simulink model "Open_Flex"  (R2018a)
settings: Solver=VariableStepAuto  StartTime=0.0  StopTime=25  FixedStep=0.0001  RelTol=1e-5  EnableMultiTasking=on
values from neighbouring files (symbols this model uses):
  d2r = pi/180    (= 0.0174532925199)    [init.m]    (also in LQR_Design.m)
  Kr = Kq; Kr(3:4)=-Kq(3:4)    [init.m]
  Wf = 24    [init.m]
undefined symbols (not defined in the file or in its folder): Aa, Av, Ba, Bv, Ca, Cv, Da, Dv, Kq, TVC

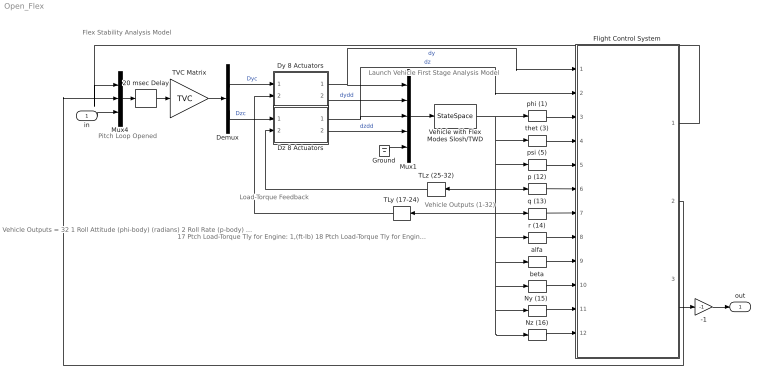
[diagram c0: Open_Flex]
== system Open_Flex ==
  note: Load-Torque Feedback
  note: 17 Ptch Load-Torque Tly for Engine: 1,(ft-lb) 18 Ptch Load-Torque Tly for Engine: 2,(ft-lb) 19 Ptch Load-Torque Tly for Engine: 3,(ft-lb) 20 Ptch Load-Torque Tly for Engine: 4,(ft-lb) 21 Ptch Load-Torque Tly for Engine: 5,(ft-lb) 22 Ptch Load-Torque Tly for Engine: 6,(ft-lb) 23 Ptch Load-Torque Tly for Engine: 7,(ft-lb) 24 Ptch Load-Torque Tly for Engine: 8,(ft-lb) 25 Yaw Load-Torque Tlz for Engine: 1,(ft-lb) 26 Yaw Load-Torque Tlz for Engine: 2,(ft-lb) 27 Yaw Load-Torque Tlz for Engine: 3,(ft-lb) 28 Yaw Load-Torque Tlz for Engine: 4,(ft-lb) 29 Yaw Load-Torque Tlz for Engine: 5,(ft-lb) 30 Yaw Load-Torque Tlz for Engine: 6,(ft-lb) 31 Yaw Load-Torque Tlz for Engine: 7,(ft-lb) 32 Yaw Load-Torque Tlz for Engine: 8,(ft-lb)
  note: Vehicle Outputs = 32 1 Roll Attitude (phi-body) (radians) 2 Roll Rate (p-body) (rad/sec) 3 Pitch Attitude (thet-bdy) (radians) 4 Pitch Rate (q-body) (rad/sec) 5 Yaw Attitude (psi-body) (radians) 6 Yaw Rate (r-body) (rad/sec) 7 Angle of attack, alfa, (radians) 8 Angle of sideslip, beta, (radian) 9 Change in Altitude, delta-h, (feet) 10 Forward Acceleration (V-dot) (ft/sec) 11 Cross Range Velocity (Vcr) (ft/sec) 12 Rate-Gyro # 1, Roll Rate (Body) (rad/sec) 13 Rate-Gyro # 2, Pitch Rate (Body) (rad/sec) 14 Rate-Gyro # 3, Yaw Rate (Body) (rad/sec) 15 Accelerom # 1, (along Y), (ft/sec^2) Translat. Accelerat. 16 Accelerom # 2, (along Z), (ft/sec^2) Translat. Accelerat.
  note: Vehicle Outputs (1-32)
  note: Flex Stability Analysis Model
  note: Pitch Loop Opened
  note: Launch Vehicle First Stage Analysis Model
  in : Inport
  -1 : Gain  Gain=-1
  20 msec Delay : TransportDelay  DelayTime="[1  1  1]*0.02"  InitialOutput="[0  0  0]"  PadeOrder=2
  Demux : Demux  Outputs=[8, 8]
  Dy 8 Actuators : Subsystem
  Dz 8 Actuators : Subsystem
  Flight Control System : Subsystem
  Ground : Ground
  Mux1 : Mux  Inputs=[8, 8, 8, 8, 1]
  Mux4 : Mux  Inputs=3
  "Ny (15) " : Selector  InputPortWidth=32  IndexOptions=Index vector (dialog)  Indices=[15]  OutputSizes=1
  Nz (16) : Selector  InputPortWidth=32  IndexOptions=Index vector (dialog)  Indices=[16]  OutputSizes=1
  TLy (17-24) : Selector  InputPortWidth=32  IndexOptions=Index vector (dialog)  Indices=[17:24]  OutputSizes=1
  TLz (25-32) : Selector  InputPortWidth=32  IndexOptions=Index vector (dialog)  Indices=[25:32]  OutputSizes=1
  TVC Matrix : Gain  Gain=TVC  Multiplication=Matrix(K*u)
  Vehicle with Flex Modes Slosh/TWD : StateSpace  A=Av  B=Bv  C=Cv  D=Dv  InitialCondition=0
  alfa : Selector  InputPortWidth=32  IndexOptions=Index vector (dialog)  Indices=[7]  OutputSizes=1
  beta : Selector  InputPortWidth=32  IndexOptions=Index vector (dialog)  Indices=[8]  OutputSizes=1
  p (12) : Selector  InputPortWidth=32  IndexOptions=Index vector (dialog)  Indices=[12]  OutputSizes=1
  phi (1) : Selector  InputPortWidth=32  IndexOptions=Index vector (dialog)  Indices=[1]  OutputSizes=1
  psi (5) : Selector  InputPortWidth=32  IndexOptions=Index vector (dialog)  Indices=[5]  OutputSizes=1
  q (13) : Selector  InputPortWidth=32  IndexOptions=Index vector (dialog)  Indices=[13]  OutputSizes=1
  r (14) : Selector  InputPortWidth=32  IndexOptions=Index vector (dialog)  Indices=[14]  OutputSizes=1
  thet (3) : Selector  InputPortWidth=32  IndexOptions=Index vector (dialog)  Indices=[3]  OutputSizes=1
  out : Outport
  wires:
  Mux1/1 -> Vehicle with Flex Modes Slosh/TWD/1
  Dy 8 Actuators/2(dydd) -> Mux1/2  "dydd"
  Dz 8 Actuators/2(dzdd) -> Mux1/4  "dzdd"
  Demux/1 -> Dy 8 Actuators/1(dyc)  "Dyc"
  Dy 8 Actuators/1(dy) -> Flight Control System/1(dy), Mux1/1  "dy"
  Dz 8 Actuators/1(dz) -> Flight Control System/2(dz), Mux1/3  "dz"
  Demux/2 -> Dz 8 Actuators/1(dzc)  "Dzc"
  TLy (17-24)/1 -> Dy 8 Actuators/2(TLy)
  TLz (25-32)/1 -> Dz 8 Actuators/2(TLz)
  Vehicle with Flex Modes Slosh/TWD/1 -> "Ny (15) "/1, Nz (16)/1, beta/1, alfa/1, r (14)/1, TLy (17-24)/1, q (13)/1, TLz (25-32)/1, p (12)/1, psi (5)/1, thet (3)/1, phi (1)/1
  r (14)/1 -> Flight Control System/8(r)
  q (13)/1 -> Flight Control System/7(q)
  p (12)/1 -> Flight Control System/6(p)
  alfa/1 -> Flight Control System/9(alfa)
  beta/1 -> Flight Control System/10(beta)
  "Ny (15) "/1 -> Flight Control System/11(NY)
  Nz (16)/1 -> Flight Control System/12(NZ)
  phi (1)/1 -> Flight Control System/3(phi)
  thet (3)/1 -> Flight Control System/4(thet)
  psi (5)/1 -> Flight Control System/5(psi)
  TVC Matrix/1 -> Demux/1
  Mux4/1 -> 20 msec Delay/1
  -1/1 -> out/1
  Ground/1 -> Mux1/5
  20 msec Delay/1 -> TVC Matrix/1
  Flight Control System/1(DP_tvc) -> Mux4/1
  Flight Control System/3(DR_tvc) -> -1/1
  in/1 -> Mux4/3
  Flight Control System/2(DQ_tvc) -> Mux4/2

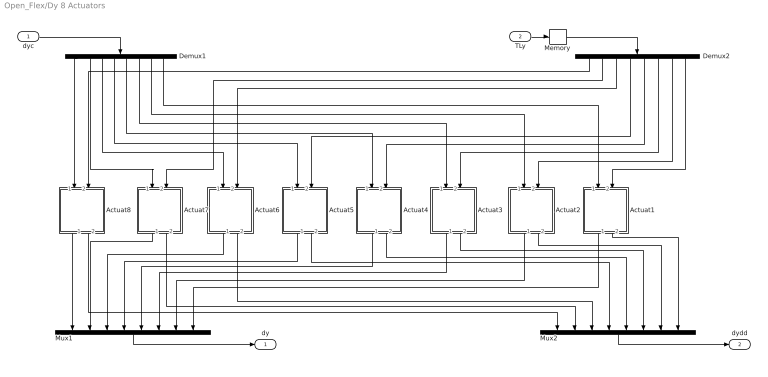
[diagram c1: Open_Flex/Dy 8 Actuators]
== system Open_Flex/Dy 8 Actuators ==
  dyc : Inport
  TLy : Inport  Port=2
  Actuat1 : Subsystem
  Actuat2 : Subsystem
  Actuat3 : Subsystem
  Actuat4 : Subsystem
  Actuat5 : Subsystem
  Actuat6 : Subsystem
  Actuat7 : Subsystem
  Actuat8 : Subsystem
  Demux1 : Demux  Outputs=8
  Demux2 : Demux  Outputs=8
  Memory : Memory
  Mux1 : Mux  Inputs=8
  Mux2 : Mux  Inputs=8
  dy : Outport
  dydd : Outport  Port=2
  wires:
  Memory/1 -> Demux2/1
  Demux1/6 -> Actuat3/1(delin)
  Actuat6/1(dout) -> Mux1/3
  Actuat3/1(dout) -> Mux1/6
  Demux2/3 -> Actuat6/2(TL)
  Demux2/8 -> Actuat1/2(TL)
  Actuat2/1(dout) -> Mux1/7
  Demux2/1 -> Actuat8/2(TL)
  Demux1/1 -> Actuat8/1(delin)
  Demux2/5 -> Actuat4/2(TL)
  Actuat7/1(dout) -> Mux1/2
  Demux1/8 -> Actuat1/1(delin)
  Demux1/7 -> Actuat2/1(delin)
  Demux1/2 -> Actuat7/1(delin)
  Actuat7/2(ddot) -> Mux2/2
  Actuat1/2(ddot) -> Mux2/8
  Mux1/1 -> dy/1
  dyc/1 -> Demux1/1
  Actuat8/2(ddot) -> Mux2/1
  Actuat2/2(ddot) -> Mux2/7
  Demux1/3 -> Actuat6/1(delin)
  Actuat5/2(ddot) -> Mux2/4
  Demux2/2 -> Actuat7/2(TL)
  Actuat6/2(ddot) -> Mux2/3
  Demux2/7 -> Actuat2/2(TL)
  Demux2/6 -> Actuat3/2(TL)
  Demux2/4 -> Actuat5/2(TL)
  Actuat4/1(dout) -> Mux1/5
  Actuat4/2(ddot) -> Mux2/5
  Actuat1/1(dout) -> Mux1/8
  Demux1/4 -> Actuat5/1(delin)
  Actuat8/1(dout) -> Mux1/1
  Actuat3/2(ddot) -> Mux2/6
  Demux1/5 -> Actuat4/1(delin)
  Actuat5/1(dout) -> Mux1/4
  Mux2/1 -> dydd/1
  TLy/1 -> Memory/1

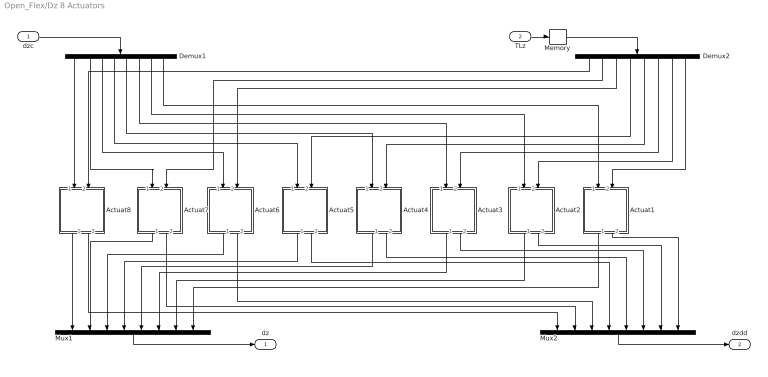
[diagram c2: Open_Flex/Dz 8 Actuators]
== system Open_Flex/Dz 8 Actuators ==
  dzc : Inport
  TLz : Inport  Port=2
  Actuat1 : Subsystem
  Actuat2 : Subsystem
  Actuat3 : Subsystem
  Actuat4 : Subsystem
  Actuat5 : Subsystem
  Actuat6 : Subsystem
  Actuat7 : Subsystem
  Actuat8 : Subsystem
  Demux1 : Demux  Outputs=8
  Demux2 : Demux  Outputs=8
  Memory : Memory
  Mux1 : Mux  Inputs=8
  Mux2 : Mux  Inputs=8
  dz : Outport
  dzdd : Outport  Port=2
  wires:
  Memory/1 -> Demux2/1
  Demux1/6 -> Actuat3/1(delin)
  Actuat6/1(dout) -> Mux1/3
  Actuat3/1(dout) -> Mux1/6
  Demux2/3 -> Actuat6/2(TL)
  Demux2/8 -> Actuat1/2(TL)
  Actuat2/1(dout) -> Mux1/7
  Demux2/1 -> Actuat8/2(TL)
  Demux1/1 -> Actuat8/1(delin)
  Demux2/5 -> Actuat4/2(TL)
  Actuat7/1(dout) -> Mux1/2
  Demux1/8 -> Actuat1/1(delin)
  Demux1/7 -> Actuat2/1(delin)
  Demux1/2 -> Actuat7/1(delin)
  Actuat7/2(ddot) -> Mux2/2
  Actuat1/2(ddot) -> Mux2/8
  Mux1/1 -> dz/1
  dzc/1 -> Demux1/1
  Actuat8/2(ddot) -> Mux2/1
  Actuat2/2(ddot) -> Mux2/7
  Demux1/3 -> Actuat6/1(delin)
  Actuat5/2(ddot) -> Mux2/4
  Demux2/2 -> Actuat7/2(TL)
  Actuat6/2(ddot) -> Mux2/3
  Demux2/7 -> Actuat2/2(TL)
  Demux2/6 -> Actuat3/2(TL)
  Demux2/4 -> Actuat5/2(TL)
  Actuat4/1(dout) -> Mux1/5
  Actuat4/2(ddot) -> Mux2/5
  Actuat1/1(dout) -> Mux1/8
  Demux1/4 -> Actuat5/1(delin)
  Actuat8/1(dout) -> Mux1/1
  Actuat3/2(ddot) -> Mux2/6
  Demux1/5 -> Actuat4/1(delin)
  Actuat5/1(dout) -> Mux1/4
  Mux2/1 -> dzdd/1
  TLz/1 -> Memory/1

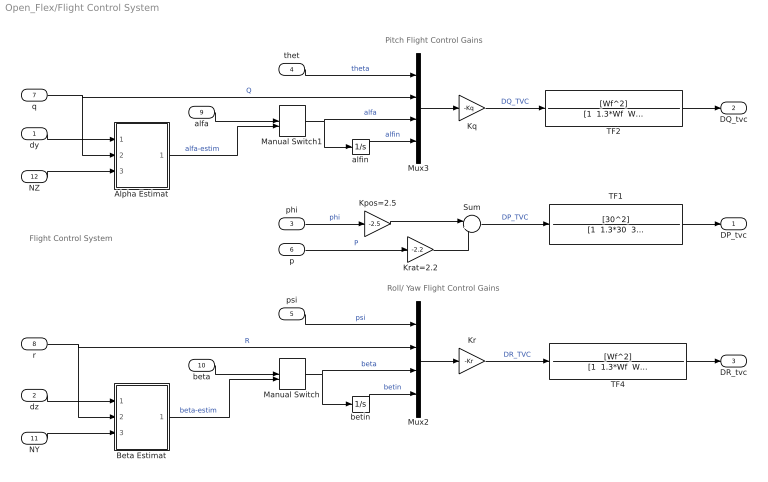
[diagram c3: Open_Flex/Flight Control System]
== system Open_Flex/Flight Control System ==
  note: Pitch Flight Control Gains
  note: Roll/ Yaw Flight Control Gains
  note: Flight Control System
  dy : Inport
  dz : Inport  Port=2
  phi : Inport  Port=3
  thet : Inport  Port=4
  psi : Inport  Port=5
  p : Inport  Port=6
  q : Inport  Port=7
  r : Inport  Port=8
  alfa : Inport  Port=9
  beta : Inport  Port=10
  NY : Inport  Port=11
  NZ : Inport  Port=12
  Alpha Estimat : Subsystem
  Beta Estimat : Subsystem
  Kpos=2.5 : Gain  Gain=-2.5  Multiplication=Matrix(K*u)
  Kq : Gain  Gain=-Kq  Multiplication=Matrix(K*u)
  Kr : Gain  Gain=-Kr  Multiplication=Matrix(K*u)
  Krat=2.2 : Gain  Gain=-2.2  Multiplication=Matrix(K*u)
  Manual Switch : ManualSwitch  CurrentSetting=0
  Manual Switch1 : ManualSwitch  CurrentSetting=0
  Mux2 : Mux
  Mux3 : Mux
  Sum : Sum  Inputs=|++
  TF1 : TransferFcn  Numerator=[30^2]  Denominator="[1  1.3*30  30^2]"
  TF2 : TransferFcn  Numerator=[Wf^2]  Denominator="[1  1.3*Wf  Wf^2]"
  TF4 : TransferFcn  Numerator=[Wf^2]  Denominator="[1  1.3*Wf  Wf^2]"
  alfin : Integrator
  betin : Integrator
  DP_tvc : Outport
  DQ_tvc : Outport  Port=2
  DR_tvc : Outport  Port=3
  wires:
  Alpha Estimat/1(alfest) -> Manual Switch1/2  "alfa-estim"
  alfa/1 -> Manual Switch1/1
  Manual Switch1/1 -> Mux3/3, alfin/1  "alfa"
  beta/1 -> Manual Switch/1
  Manual Switch/1 -> betin/1, Mux2/3  "beta"
  psi/1 -> Mux2/1  "psi"
  betin/1 -> Mux2/4  "betin"
  q/1 -> Alpha Estimat/2(q), Mux3/2  "Q"
  r/1 -> Beta Estimat/2(r), Mux2/2  "R"
  alfin/1 -> Mux3/4  "alfin"
  Kr/1 -> TF4/1  "DR_TVC"
  thet/1 -> Mux3/1  "theta"
  Kq/1 -> TF2/1  "DQ_TVC"
  TF4/1 -> DR_tvc/1
  TF2/1 -> DQ_tvc/1
  NZ/1 -> Alpha Estimat/3(Zdd)
  NY/1 -> Beta Estimat/3(Ydd)
  Beta Estimat/1(betest) -> Manual Switch/2  "beta-estim"
  dy/1 -> Alpha Estimat/1(dy)
  dz/1 -> Beta Estimat/1(dz)
  Mux3/1 -> Kq/1
  Kpos=2.5/1 -> Sum/1
  Sum/1 -> TF1/1  "DP_TVC"
  Krat=2.2/1 -> Sum/2
  p/1 -> Krat=2.2/1  "P"
  phi/1 -> Kpos=2.5/1  "phi"
  Mux2/1 -> Kr/1
  TF1/1 -> DP_tvc/1

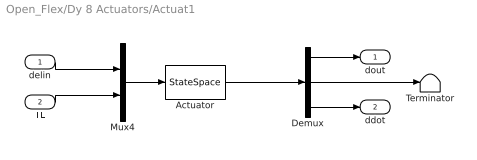
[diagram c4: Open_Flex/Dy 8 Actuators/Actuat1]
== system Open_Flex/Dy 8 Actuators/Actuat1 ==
  delin : Inport
  TL : Inport  Port=2
  Actuator : StateSpace  A=Aa  B=Ba  C=Ca  D=Da  InitialCondition=0
  Demux : Demux  Outputs=3
  Mux4 : Mux  Inputs=2
  Terminator : Terminator
  dout : Outport
  ddot : Outport  Port=2
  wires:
  Demux/2 -> Terminator/1
  Demux/1 -> dout/1
  delin/1 -> Mux4/1
  Actuator/1 -> Demux/1
  Mux4/1 -> Actuator/1
  TL/1 -> Mux4/2
  Demux/3 -> ddot/1

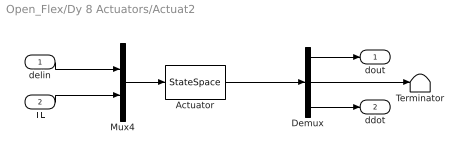
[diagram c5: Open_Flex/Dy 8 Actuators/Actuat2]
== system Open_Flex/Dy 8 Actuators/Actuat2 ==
  delin : Inport
  TL : Inport  Port=2
  Actuator : StateSpace  A=Aa  B=Ba  C=Ca  D=Da  InitialCondition=0
  Demux : Demux  Outputs=3
  Mux4 : Mux  Inputs=2
  Terminator : Terminator
  dout : Outport
  ddot : Outport  Port=2
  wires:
  Demux/2 -> Terminator/1
  Demux/1 -> dout/1
  delin/1 -> Mux4/1
  Actuator/1 -> Demux/1
  Mux4/1 -> Actuator/1
  TL/1 -> Mux4/2
  Demux/3 -> ddot/1

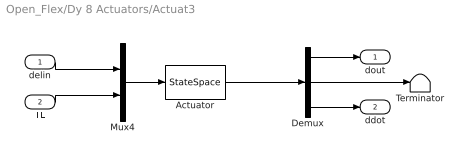
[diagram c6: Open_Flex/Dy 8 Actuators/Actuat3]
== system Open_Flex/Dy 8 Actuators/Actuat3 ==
  delin : Inport
  TL : Inport  Port=2
  Actuator : StateSpace  A=Aa  B=Ba  C=Ca  D=Da  InitialCondition=0
  Demux : Demux  Outputs=3
  Mux4 : Mux  Inputs=2
  Terminator : Terminator
  dout : Outport
  ddot : Outport  Port=2
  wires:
  Demux/2 -> Terminator/1
  Demux/1 -> dout/1
  delin/1 -> Mux4/1
  Actuator/1 -> Demux/1
  Mux4/1 -> Actuator/1
  TL/1 -> Mux4/2
  Demux/3 -> ddot/1

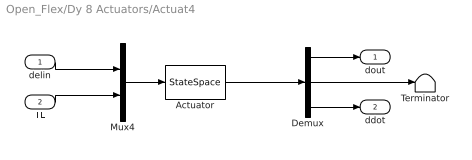
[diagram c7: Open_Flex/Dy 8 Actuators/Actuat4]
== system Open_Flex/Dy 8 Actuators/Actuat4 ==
  delin : Inport
  TL : Inport  Port=2
  Actuator : StateSpace  A=Aa  B=Ba  C=Ca  D=Da  InitialCondition=0
  Demux : Demux  Outputs=3
  Mux4 : Mux  Inputs=2
  Terminator : Terminator
  dout : Outport
  ddot : Outport  Port=2
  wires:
  Demux/2 -> Terminator/1
  Demux/1 -> dout/1
  delin/1 -> Mux4/1
  Actuator/1 -> Demux/1
  Mux4/1 -> Actuator/1
  TL/1 -> Mux4/2
  Demux/3 -> ddot/1

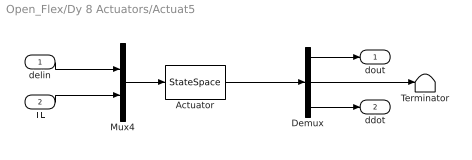
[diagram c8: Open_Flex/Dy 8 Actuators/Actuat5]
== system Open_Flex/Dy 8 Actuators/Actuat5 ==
  delin : Inport
  TL : Inport  Port=2
  Actuator : StateSpace  A=Aa  B=Ba  C=Ca  D=Da  InitialCondition=0
  Demux : Demux  Outputs=3
  Mux4 : Mux  Inputs=2
  Terminator : Terminator
  dout : Outport
  ddot : Outport  Port=2
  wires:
  Demux/2 -> Terminator/1
  Demux/1 -> dout/1
  delin/1 -> Mux4/1
  Actuator/1 -> Demux/1
  Mux4/1 -> Actuator/1
  TL/1 -> Mux4/2
  Demux/3 -> ddot/1

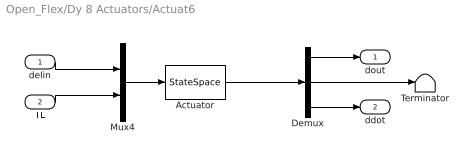
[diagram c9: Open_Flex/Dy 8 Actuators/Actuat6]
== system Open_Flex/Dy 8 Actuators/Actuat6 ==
  delin : Inport
  TL : Inport  Port=2
  Actuator : StateSpace  A=Aa  B=Ba  C=Ca  D=Da  InitialCondition=0
  Demux : Demux  Outputs=3
  Mux4 : Mux  Inputs=2
  Terminator : Terminator
  dout : Outport
  ddot : Outport  Port=2
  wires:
  Demux/2 -> Terminator/1
  Demux/1 -> dout/1
  delin/1 -> Mux4/1
  Actuator/1 -> Demux/1
  Mux4/1 -> Actuator/1
  TL/1 -> Mux4/2
  Demux/3 -> ddot/1

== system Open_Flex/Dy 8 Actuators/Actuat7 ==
  delin : Inport
  TL : Inport  Port=2
  Actuator : StateSpace  A=Aa  B=Ba  C=Ca  D=Da  InitialCondition=0
  Demux : Demux  Outputs=3
  Mux4 : Mux  Inputs=2
  Terminator : Terminator
  dout : Outport
  ddot : Outport  Port=2
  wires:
  Demux/2 -> Terminator/1
  Demux/1 -> dout/1
  delin/1 -> Mux4/1
  Actuator/1 -> Demux/1
  Mux4/1 -> Actuator/1
  TL/1 -> Mux4/2
  Demux/3 -> ddot/1

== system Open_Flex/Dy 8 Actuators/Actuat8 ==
  delin : Inport
  TL : Inport  Port=2
  Actuator : StateSpace  A=Aa  B=Ba  C=Ca  D=Da  InitialCondition=0
  Demux : Demux  Outputs=3
  Mux4 : Mux  Inputs=2
  Terminator : Terminator
  dout : Outport
  ddot : Outport  Port=2
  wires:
  Demux/2 -> Terminator/1
  Demux/1 -> dout/1
  delin/1 -> Mux4/1
  Actuator/1 -> Demux/1
  Mux4/1 -> Actuator/1
  TL/1 -> Mux4/2
  Demux/3 -> ddot/1

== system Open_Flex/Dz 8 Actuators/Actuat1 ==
  delin : Inport
  TL : Inport  Port=2
  Actuator : StateSpace  A=Aa  B=Ba  C=Ca  D=Da  InitialCondition=0
  Demux : Demux  Outputs=3
  Mux4 : Mux  Inputs=2
  Terminator : Terminator
  dout : Outport
  ddot : Outport  Port=2
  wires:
  Demux/2 -> Terminator/1
  Demux/1 -> dout/1
  delin/1 -> Mux4/1
  Actuator/1 -> Demux/1
  Mux4/1 -> Actuator/1
  TL/1 -> Mux4/2
  Demux/3 -> ddot/1

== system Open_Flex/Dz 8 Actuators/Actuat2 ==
  delin : Inport
  TL : Inport  Port=2
  Actuator : StateSpace  A=Aa  B=Ba  C=Ca  D=Da  InitialCondition=0
  Demux : Demux  Outputs=3
  Mux4 : Mux  Inputs=2
  Terminator : Terminator
  dout : Outport
  ddot : Outport  Port=2
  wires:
  Demux/2 -> Terminator/1
  Demux/1 -> dout/1
  delin/1 -> Mux4/1
  Actuator/1 -> Demux/1
  Mux4/1 -> Actuator/1
  TL/1 -> Mux4/2
  Demux/3 -> ddot/1

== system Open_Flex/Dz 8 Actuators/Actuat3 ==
  delin : Inport
  TL : Inport  Port=2
  Actuator : StateSpace  A=Aa  B=Ba  C=Ca  D=Da  InitialCondition=0
  Demux : Demux  Outputs=3
  Mux4 : Mux  Inputs=2
  Terminator : Terminator
  dout : Outport
  ddot : Outport  Port=2
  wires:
  Demux/2 -> Terminator/1
  Demux/1 -> dout/1
  delin/1 -> Mux4/1
  Actuator/1 -> Demux/1
  Mux4/1 -> Actuator/1
  TL/1 -> Mux4/2
  Demux/3 -> ddot/1

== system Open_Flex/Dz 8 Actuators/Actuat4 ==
  delin : Inport
  TL : Inport  Port=2
  Actuator : StateSpace  A=Aa  B=Ba  C=Ca  D=Da  InitialCondition=0
  Demux : Demux  Outputs=3
  Mux4 : Mux  Inputs=2
  Terminator : Terminator
  dout : Outport
  ddot : Outport  Port=2
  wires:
  Demux/2 -> Terminator/1
  Demux/1 -> dout/1
  delin/1 -> Mux4/1
  Actuator/1 -> Demux/1
  Mux4/1 -> Actuator/1
  TL/1 -> Mux4/2
  Demux/3 -> ddot/1

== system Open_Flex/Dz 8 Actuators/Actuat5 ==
  delin : Inport
  TL : Inport  Port=2
  Actuator : StateSpace  A=Aa  B=Ba  C=Ca  D=Da  InitialCondition=0
  Demux : Demux  Outputs=3
  Mux4 : Mux  Inputs=2
  Terminator : Terminator
  dout : Outport
  ddot : Outport  Port=2
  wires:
  Demux/2 -> Terminator/1
  Demux/1 -> dout/1
  delin/1 -> Mux4/1
  Actuator/1 -> Demux/1
  Mux4/1 -> Actuator/1
  TL/1 -> Mux4/2
  Demux/3 -> ddot/1

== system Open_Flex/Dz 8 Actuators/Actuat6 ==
  delin : Inport
  TL : Inport  Port=2
  Actuator : StateSpace  A=Aa  B=Ba  C=Ca  D=Da  InitialCondition=0
  Demux : Demux  Outputs=3
  Mux4 : Mux  Inputs=2
  Terminator : Terminator
  dout : Outport
  ddot : Outport  Port=2
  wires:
  Demux/2 -> Terminator/1
  Demux/1 -> dout/1
  delin/1 -> Mux4/1
  Actuator/1 -> Demux/1
  Mux4/1 -> Actuator/1
  TL/1 -> Mux4/2
  Demux/3 -> ddot/1

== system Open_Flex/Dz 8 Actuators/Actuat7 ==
  delin : Inport
  TL : Inport  Port=2
  Actuator : StateSpace  A=Aa  B=Ba  C=Ca  D=Da  InitialCondition=0
  Demux : Demux  Outputs=3
  Mux4 : Mux  Inputs=2
  Terminator : Terminator
  dout : Outport
  ddot : Outport  Port=2
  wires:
  Demux/2 -> Terminator/1
  Demux/1 -> dout/1
  delin/1 -> Mux4/1
  Actuator/1 -> Demux/1
  Mux4/1 -> Actuator/1
  TL/1 -> Mux4/2
  Demux/3 -> ddot/1

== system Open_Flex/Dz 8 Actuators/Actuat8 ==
  delin : Inport
  TL : Inport  Port=2
  Actuator : StateSpace  A=Aa  B=Ba  C=Ca  D=Da  InitialCondition=0
  Demux : Demux  Outputs=3
  Mux4 : Mux  Inputs=2
  Terminator : Terminator
  dout : Outport
  ddot : Outport  Port=2
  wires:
  Demux/2 -> Terminator/1
  Demux/1 -> dout/1
  delin/1 -> Mux4/1
  Actuator/1 -> Demux/1
  Mux4/1 -> Actuator/1
  TL/1 -> Mux4/2
  Demux/3 -> ddot/1

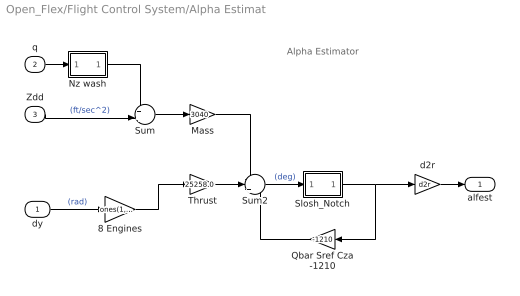
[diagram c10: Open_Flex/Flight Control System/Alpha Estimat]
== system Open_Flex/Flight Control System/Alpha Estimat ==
  note: Alpha Estimator
  dy : Inport
  q : Inport  Port=2
  Zdd : Inport  Port=3
  8 Engines : Gain  Gain=ones(1,8)  Multiplication=Matrix(K*u) (u vector)
  Mass : Gain  Gain=3040
  Nz wash : Subsystem
  Qbar Sref Cza -1210 : Gain  Gain=-1210
  Slosh_Notch : Subsystem
  Sum : Sum  Inputs=++|
  Sum2 : Sum  Inputs=--+
  Thrust : Gain  Gain=25258.0
  d2r : Gain  Gain=d2r
  alfest : Outport
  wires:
  8 Engines/1 -> Thrust/1
  Thrust/1 -> Sum2/2
  Mass/1 -> Sum2/1
  Slosh_Notch/1(ou) -> Qbar Sref Cza -1210/1, d2r/1
  Nz wash/1(ou) -> Sum/1
  Sum2/1 -> Slosh_Notch/1(in)  "(deg)"
  Qbar Sref Cza -1210/1 -> Sum2/3
  Zdd/1 -> Sum/2  "(ft/sec^2)"
  d2r/1 -> alfest/1
  q/1 -> Nz wash/1(in)
  Sum/1 -> Mass/1
  dy/1 -> 8 Engines/1  "(rad)"

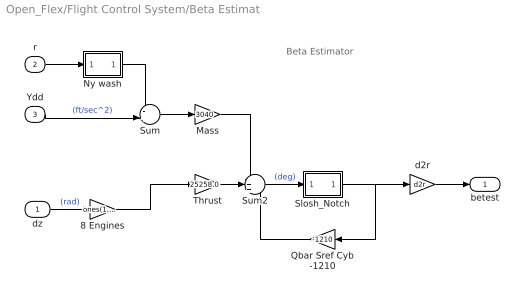
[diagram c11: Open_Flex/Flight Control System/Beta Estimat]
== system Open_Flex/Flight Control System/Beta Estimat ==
  note: Beta Estimator
  dz : Inport
  r : Inport  Port=2
  Ydd : Inport  Port=3
  8 Engines : Gain  Gain=ones(1,8)  Multiplication=Matrix(K*u) (u vector)
  Mass : Gain  Gain=3040
  Ny wash : Subsystem
  Qbar Sref Cyb -1210 : Gain  Gain=-1210
  Slosh_Notch : Subsystem
  Sum : Sum  Inputs=-+|
  Sum2 : Sum  Inputs=-++
  Thrust : Gain  Gain=25258.0
  d2r : Gain  Gain=d2r
  betest : Outport
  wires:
  8 Engines/1 -> Thrust/1
  dz/1 -> 8 Engines/1  "(rad)"
  Slosh_Notch/1(ou) -> d2r/1, Qbar Sref Cyb -1210/1
  Ny wash/1(ou) -> Sum/1
  Sum2/1 -> Slosh_Notch/1(in)  "(deg)"
  Qbar Sref Cyb -1210/1 -> Sum2/3
  Ydd/1 -> Sum/2  "(ft/sec^2)"
  Mass/1 -> Sum2/1
  d2r/1 -> betest/1
  Thrust/1 -> Sum2/2
  r/1 -> Ny wash/1(in)
  Sum/1 -> Mass/1

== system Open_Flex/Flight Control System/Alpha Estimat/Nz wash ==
  in : Inport
  3 : Gain  Gain=19
  Transfer Fcn : TransferFcn  Numerator="[1  0]"  Denominator="[0.015  1]"
  ou : Outport
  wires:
  3/1 -> ou/1
  Transfer Fcn/1 -> 3/1
  in/1 -> Transfer Fcn/1

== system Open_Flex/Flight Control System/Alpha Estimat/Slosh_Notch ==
  in : Inport
  0.1 : Gain  Gain=0.0004
  Int1 : Integrator
  Transfer Fcn2 : TransferFcn  Numerator="[1 0.016*5  5.12^2]"  Denominator="[1  0.38*5  5.12^2]"
  ou : Outport
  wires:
  Int1/1 -> ou/1
  in/1 -> 0.1/1
  0.1/1 -> Transfer Fcn2/1
  Transfer Fcn2/1 -> Int1/1

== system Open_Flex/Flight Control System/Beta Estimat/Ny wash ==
  in : Inport
  3 : Gain  Gain=19
  Transfer Fcn1 : TransferFcn  Numerator="[1  0]"  Denominator="[0.015  1]"
  ou : Outport
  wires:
  3/1 -> ou/1
  Transfer Fcn1/1 -> 3/1
  in/1 -> Transfer Fcn1/1

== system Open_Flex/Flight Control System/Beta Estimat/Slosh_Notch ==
  in : Inport
  0.1 : Gain  Gain=0.0004
  Int1 : Integrator
  Transfer Fcn1 : TransferFcn  Numerator="[1 0.016*5  5.12^2]"  Denominator="[1  0.38*5  5.12^2]"
  ou : Outport
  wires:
  Transfer Fcn1/1 -> Int1/1
  0.1/1 -> Transfer Fcn1/1
  Int1/1 -> ou/1
  in/1 -> 0.1/1
